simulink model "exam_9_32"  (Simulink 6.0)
settings: Solver=ode45  StartTime=0.0  StopTime=10.0  RelTol=1e-3

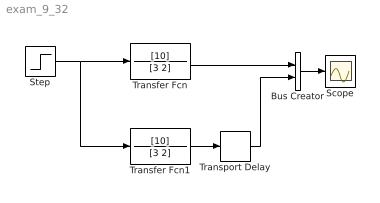
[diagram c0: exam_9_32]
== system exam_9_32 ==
  Bus Creator : BusCreator  DialogController=Simulink.DDGSource_Bus  Inputs=2
  Scope : Scope
  Step : Step  SampleTime=0
  Transfer Fcn : TransferFcn  Numerator=[10]  Denominator=[3 2]
  Transfer Fcn1 : TransferFcn  Numerator=[10]  Denominator=[3 2]
  Transport Delay : TransportDelay
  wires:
  Bus Creator/1 -> Scope/1
  Transfer Fcn1/1 -> Transport Delay/1
  Transport Delay/1 -> Bus Creator/2
  Transfer Fcn/1 -> Bus Creator/1
  Step/1 -> Transfer Fcn/1, Transfer Fcn1/1
